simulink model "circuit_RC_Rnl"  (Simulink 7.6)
settings: Solver=ode15s  StartTime=0.0  StopTime=0.12  RelTol=1e-3
InitFcn:
  | clc
StopFcn:
  | close all
  | load UI_circuit_RC.mat
  | plotyy(ui(1,:),ui(2,:),ui(1,:),ui(3,:))
  | 
  | title('Tension aux bornes de C et courant dans le circuit RC, avec R non linéaire')
  | xlabel('temps')
  | grid
  | 
  | % Tracé de la résistance
  | u=ui(4,:)-ui(3,:);
  | i=ui(2,:);
  | 
  | R=u./i;
  | figure
  | plot(ui(1,:),R)
  | grid
  | title('Evolution de la résistance en Ohm')
  | xlabel('temps')
libraries: fl_lib x5, nesl_utility x4, MaLibrairieElectrical_lib x1

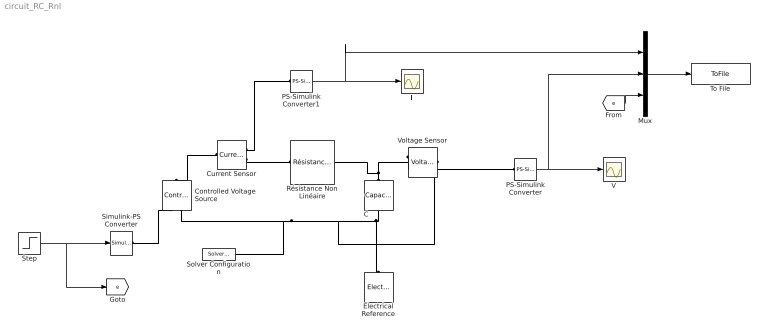
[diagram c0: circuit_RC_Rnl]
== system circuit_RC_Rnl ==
  C : fl_lib/Electrical/Electrical Elements/Capacitor  DialogController=NetworkEngine.DynNeDlgSource  SystemSampleTime=-1  c=1e-3 F  v0=0 V  r=1e-6 Ohm  g=0 1/Ohm  i_Log=off  v_Log=off  vc_Log=off  LocalVarNames=|i|v|vc  LocalVarDescs=|i|v|Internal variable for voltage across capacitor term  LocalVarLogging=[0 0 0]
  Controlled Voltage Source : fl_lib/Electrical/Electrical Sources/Controlled Voltage Source  DialogController=NetworkEngine.DynNeDlgSource  SystemSampleTime=-1  i_Log=off  v_Log=off  LocalVarNames=|i|v  LocalVarDescs=|i|v  LocalVarLogging=[0 0]
  Current Sensor : fl_lib/Electrical/Electrical Sensors/Current Sensor  DialogController=NetworkEngine.DynNeDlgSource  SystemSampleTime=-1  i1_Log=off  v1_Log=off  LocalVarNames=|i1|v1  LocalVarDescs=|i1|v1  LocalVarLogging=[0 0]
  Electrical Reference : fl_lib/Electrical/Electrical Elements/Electrical Reference  DialogController=NetworkEngine.DynNeDlgSource  SystemSampleTime=-1  i_Log=off  LocalVarNames=|i  LocalVarDescs=|i  LocalVarLogging=0
  I : Scope
  Mux : Mux  Inputs=3
  PS-Simulink Converter : nesl_utility/PS-Simulink Converter  DialogController=NetworkEngine.DynNeUtilDlgSource  SystemSampleTime=-1  PhysicalDomain=network_engine_domain  LeftPortType=input  RightPortType=output  SubClassName=ps_output  Unit=1  AffineConversion=off
  PS-Simulink Converter1 : nesl_utility/PS-Simulink Converter  DialogController=NetworkEngine.DynNeUtilDlgSource  SystemSampleTime=-1  PhysicalDomain=network_engine_domain  LeftPortType=input  RightPortType=output  SubClassName=ps_output  Unit=1  AffineConversion=off
  Résistance Non Linéaire : MaLibrairieElectrical_lib/Résistance Non Linéaire  DialogController=NetworkEngine.DynNeDlgSource  SystemSampleTime=-1  K=100 V/A^2  v_Log=off  i_Log=off  LocalVarNames=|v|i  LocalVarDescs=|v|i  LocalVarLogging=[0 0]
  Simulink-PS Converter : nesl_utility/Simulink-PS Converter  DialogController=NetworkEngine.DynNeUtilDlgSource  SystemSampleTime=-1  PhysicalDomain=network_engine_domain  LeftPortType=input  RightPortType=output  SubClassName=ps_input  Unit=1  AffineConversion=off  InputFilterTimeConstant=.001  UdotUserProvided=0
  Solver Configuration : nesl_utility/Solver Configuration  DialogController=NetworkEngine.DynNeUtilDlgSource  SystemSampleTime=-1  PhysicalDomain=network_engine_domain  LeftPortType=input  RightPortType=generic  SubClassName=solver  Accelerate=off  Profile=off  ResidualTolerance=1e-9  MaxNonlinIter=3  MaxModeIter=2  DoFixedCost=off  UseLocalSampling=off  DoDC=off  LinearAlgebra=Sparse  LocalSolverSampleTime=.001  LocalSolverChoice=NE_BACKWARD_EULER_ADVANCER  UseLocalSolver=off
  Step : Step  Time=0  After=12  SampleTime=0
  To File : ToFile  Filename=UI_circuit_RC  MatrixName=ui
  V : Scope
  Voltage Sensor : fl_lib/Electrical/Electrical Sensors/Voltage Sensor  DialogController=NetworkEngine.DynNeDlgSource  SystemSampleTime=-1  i1_Log=off  v1_Log=off  LocalVarNames=|i1|v1  LocalVarDescs=|i1|v1  LocalVarLogging=[0 0]
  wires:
  Step/1 -> Simulink-PS Converter/1, [e]
  PS-Simulink Converter/1 -> V/1, Mux/2
  PS-Simulink Converter1/1 -> I/1, Mux/1
  Mux/1 -> To File/1
  [e] -> Mux/3
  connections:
  Controlled Voltage Source/RConn2 -- C/RConn1 -- Electrical Reference/LConn1 -- Voltage Sensor/RConn2 -- Solver Configuration/RConn1
  C/LConn1 -- Voltage Sensor/LConn1 -- Résistance Non Linéaire/RConn1
  Simulink-PS Converter/RConn1 -- Controlled Voltage Source/RConn1
  Voltage Sensor/RConn1 -- PS-Simulink Converter/LConn1
  Current Sensor/LConn1 -- Controlled Voltage Source/LConn1
  Current Sensor/RConn1 -- PS-Simulink Converter1/LConn1
  Current Sensor/RConn2 -- Résistance Non Linéaire/LConn1
